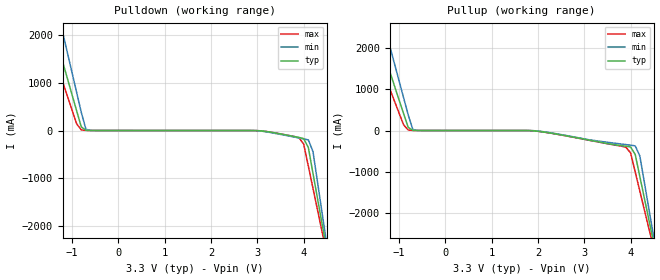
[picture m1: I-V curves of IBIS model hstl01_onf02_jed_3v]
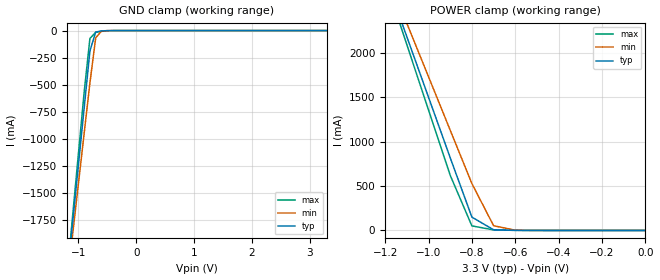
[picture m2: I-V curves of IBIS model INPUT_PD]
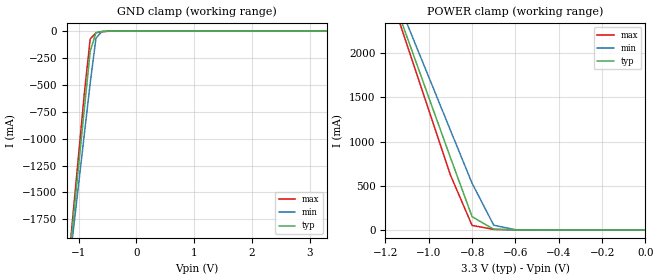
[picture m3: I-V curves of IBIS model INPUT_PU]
|   This file is an IBIS representation of the   |
|   Integrated Circuit Systems, Inc.   |
|   ICS85211i_01   |
|   Differential to HSTL Translator   |
[IBIS Ver]   3.2
[File name]   85211i_01_3v.ibs
[File Rev]   1.0
[Date]   Apr 2 2004 | Last modified
|   Apr 31 2004 | Generated
[Source] Originated at Integrated Circuit Systems, Inc.
[Disclaimer]
ICS hereby grants the user of this IBIS model a non-exclusive,
nontransferable license to use this IBIS model under the following terms.
Before using this IBIS model, the user should read this license.
If the user does not accept these terms,  the IBIS model should be
returned to ICS within 30 days.
   The user is granted this license only to use the IBIS model and
is not granted rights to sell, load, rent, lease or license the IBIS
model in whole or in part, or in modified form to anyone other than
user. User may modify the IBIS model to suit its specific
applications but rights to derivative works and such modifications
shall belong to ICS.
   This IBIS model is provided on an "AS IS" basis and ICS makes
absolutely no warranty with respect to the information contained
herein. ICS DISCLAIMS AND CUSTOMER WAIVES ALL WARRANTIES, EXPRESS
OR IMPLIED, INCLUDING WARRANTIES OF MERCHANTABILITY OR FITNESS FOR
A PARTICULAR PURPOSE. The entire risk as to quality and performance
is with the Customer. ACCORDINGLY, IN NO EVENT SHALL THE COMPANY BE
LIABLE FOR ANY DAMAGES, WHETHER IN CONTRACT OR TORT,INCLUDING ANY
LOST PROFITS OR OTHER INCIDENTAL, CONSEQUENTIAL, EXEMPLARY, OR
PUNITIVE DAMAGES ARISING OUT OF THE USE OR APPLICATION OF THE IBIS
model provided in this package. Further, ICS reserves the right to
make changes without notice to any product herein to improve
reliability, function, or design. ICS does not convey any license
under patent rights or any other intellectual property rights,
including those of third parties.
   ICS is not obligated to provide maintenance or support
for the licensed IBIS model.
[Copyright]   Copyright 2004 by Integrated Circuit Systems, Inc.
[Component]   ICS85211i_01
[Manufacturer] Integrated Circuit Systems, Inc.
[Package]
|SOIC 8 Lead
|   typ   min   max
R_pkg   57.05m   55.5m   58.6m
L_pkg   1.769nH   1.570nH   1.968nH
C_pkg   0.269pF   0.252pF   0.286pF
[Pin] signal_name   model_name
1   Q0   hstl01_onf02_jed_3v
2   nQ0   hstl01_onf02_jed_3v
3   Q1   hstl01_onf02_jed_3v
4   nQ1   hstl01_onf02_jed_3v
5   GND   GND
6   nCLK   INPUT_PD
7   CLK   INPUT_PU
8   VDD   Power
[Diff Pin]  inv_pin  vdiff tdelay_typ tdelay_min  tdelay_max
1   2   NA   0  0  0
3   4   NA   0  0  0
| Models and submodels in the file (3): hstl01_onf02_jed_3v (Output_ECL), INPUT_PD (Input), INPUT_PU (Input)
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[Model]   hstl01_onf02_jed_3v
Model_type  Output_ECL
Polarity   Non-Inverting
|Variable   typ   min   max
C_comp   2p   1.5p   2.5p
[Voltage Range]   3.3V   3.135V   3.465V
|  Voltage   I(typ)   I(min)   I(max)
[Pullup]
-3.3V     8.641A     10.88A     7.185A
-1.7V     3.146A     4.15A      2.48A
-1.5V     2.46A      3.31A      1.893A
-1.3V     1.776A     2.471A     1.307A
-800mV    75.74mA    379.7mA    12.36mA
-600mV    1.036mA    1.13mA     1.172mA
2V        -17.52mA   -12.22mA   -18.15mA
4V        -397.8mA   -353.5mA   -540.4mA
4.2V      -1.114A    -616.1mA   -1.465A
4.4V      -2.185A    -1.927A    -2.39A
4.5V      -2.72A     -2.582A    -2.848A
6.6V      -13.98A    -16.37A    -12.49A
[Pulldown]
-3.3V     8.641A     10.88A     7.185A
-1.6V     2.803A     3.73A      2.186A
-1.4V     2.118A     2.891A     1.6A
-1.2V     1.434A     2.052A     1.015A
-800mV    75.74mA    379.7mA    12.36mA
-600mV    1.036mA    1.13mA     1.172mA
3.9V      -145.6mA   -156.8mA   -152.4mA
4.1V      -356.7mA   -196.4mA   -747.5mA
4.2V      -897.6mA   -441.3mA   -1.212A
4.4V      -1.98A     -1.752A    -2.141A
4.5V      -2.521A    -2.407A    -2.606A
6.6V      -13.86A    -16.27A    -12.36A
[Ramp]
|   typ   min   max
dV/dt_r   0.6V/0.5ns   0.6V/0.6ns   0.6V/0.4ns
dV/dt_f   0.6V/0.4ns   0.6V/0.5ns   0.6V/0.3ns
R_load =   50.0000
[Model]   INPUT_PD
Model_type   Input
Polarity   Non-Inverting
Vinl = 1.4V
Vinh = 1.85V
|   typ   min   max
C_comp   2pF   1.5pF   2.5pF
|   typ   min   max
[Voltage range]  3.3V   3.15V   3.45V
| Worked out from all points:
|   GND clamp passes 1 mA (typ) near -0.51 V on its own axis
|   POWER clamp passes 1 mA (typ) near -0.60 V on its own axis
[GND_clamp]
|Voltage I(typ)   I(min)   I(max)
-3.3V     -13.52A    -12.28A    -14.38A
-1.2V     -2.314A    -2.362A    -2.296A
-1.1V     -1.782A    -1.891A    -1.721A
-1V       -1.25A     -1.422A    -1.146A
-900mV    -718.5mA   -952.6mA   -572.1mA
-800mV    -188.2mA   -484.5mA   -72.95mA
-700mV    -13.66mA   -66.68mA   -15.82mA
-600mV    -3.044mA   -4.415mA   -6.968mA
-500mV    -658.9uA   -400.5uA   -2.169mA
3.3V      64.58uA    64.62uA    64.6uA
[POWER_clamp]
|Voltage   I(typ)   I(min)   I(max)
-3.3V     17.27A     15.67A     18.38A
-1.2V     2.866A     2.938A     2.832A
-1.1V     2.183A     2.334A     2.094A
-1V       1.501A     1.732A     1.358A
-900mV    819.8mA    1.13A      621.9mA
-800mV    150.3mA    528.4mA    51.58mA
-700mV    7.809mA    53.45mA    6.607mA
-600mV    968.4uA    3.161mA    1.955mA
0V        64.58uA    61.35uA    67.83uA
[Model]   INPUT_PU
Model_type   Input
Polarity   Non-Inverting
Vinl = 1.4V
Vinh = 1.85V
|   typ   min   max
C_comp   2pF   1.5pF   2.5pF
|   typ   min   max
[Voltage range]  3.3V   3.15V   3.45V
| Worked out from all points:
|   GND clamp passes 1 mA (typ) near -0.51 V on its own axis
|   POWER clamp passes 1 mA (typ) near -0.60 V on its own axis
[GND_clamp]
|Voltage   I(typ)   I(min)   I(max)
-3.3V     -13.52A    -12.28A    -14.38A
-1.2V     -2.314A    -2.362A    -2.296A
-1.1V     -1.782A    -1.891A    -1.721A
-1V       -1.25A     -1.422A    -1.146A
-900mV    -718.6mA   -952.7mA   -572.2mA
-800mV    -188.2mA   -484.6mA   -73.02mA
-700mV    -13.72mA   -66.74mA   -15.89mA
-600mV    -3.109mA   -4.477mA   -7.036mA
-500mV    -723.5uA   -462.1uA   -2.236mA
3.3V      3.748nA    2.972uA    -2.918uA
[POWER_clamp]
|Voltage   I(typ)   I(min)   I(max)
-3.3V     17.27A     15.67A     18.38A
-1.2V     2.866A     2.938A     2.832A
-1.1V     2.183A     2.334A     2.094A
-1V       1.501A     1.732A     1.358A
-900mV    819.7mA    1.129A     621.8mA
-800mV    150.2mA    528.4mA    51.51mA
-700mV    7.744mA    53.39mA    6.54mA
-600mV    903.9uA    3.099mA    1.887mA
0V        3.748nA    2.31nA     19.96nA
